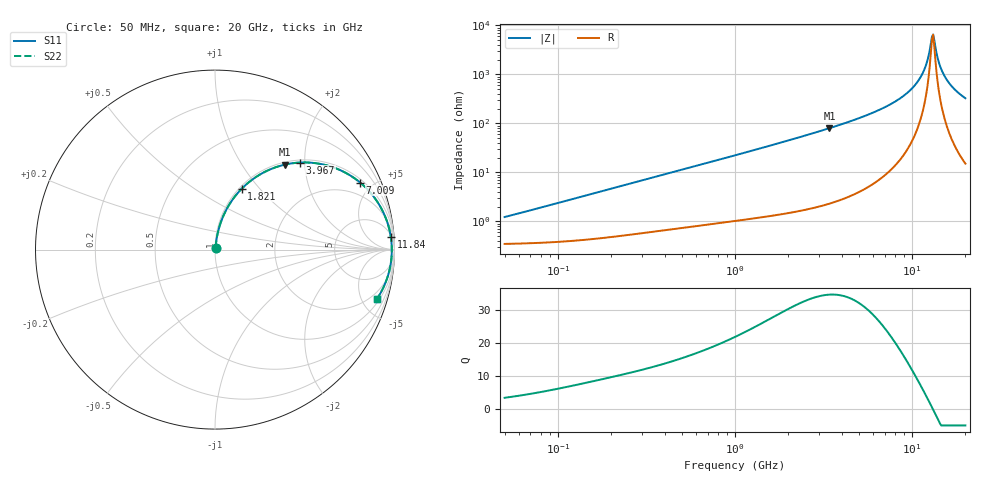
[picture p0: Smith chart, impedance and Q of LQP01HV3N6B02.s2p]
!Murata Part Number: LQP01HV3N6B02
!These Parameters are Measured in Series Mode Connection
!  o--[Z]--o
!Port1  Port2
!  o-------o
!Freq. Start=50[MHz] Stop=20[GHz], 401[Steps]
# Hz S RI R 50
!Freq.(Hz) S11(Real) S11(Imag) S21(Real) S21(Imag) S12(Real) S12(Imag) S22(Real) S22(Imag)
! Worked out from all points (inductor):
!   401 points, 50 MHz to 20 GHz, reference 50 ohm
!   read as one part in series: L = 3.72 nH near 51.52 MHz
!   highest Q = 34.7 at 3.415 GHz (marker M1), where L = 3.7 nH
!   self-resonance near 12.95 GHz
!   S11 on the Smith chart (normalised r, x): 50 MHz: 1.01, +0.02; 1.821 GHz: 1.03, +0.81; 3.967 GHz: 1.05, +1.89; 7.009 GHz: 1.17, +4.24; 11.84 GHz: 7, +27; 20 GHz: 1.30, -6.48
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5e7  0.00357 0.0116  0.9964 -0.0116  0.9964 -0.0116  0.00357 0.0116
1.364002e8  0.0051 0.0313  0.9949 -0.0313  0.9949 -0.0313  0.0051 0.0313
3.721004e8  0.0132 0.0824  0.9868 -0.0824  0.9868 -0.0824  0.0132 0.0824
1e9  0.0554 0.207  0.9446 -0.207  0.9446 -0.207  0.0554 0.207
1.820564e9  0.1492 0.3395  0.8508 -0.3395  0.8508 -0.3395  0.1492 0.3395
2.728004e9  0.283 0.4358  0.717 -0.4358  0.717 -0.4358  0.283 0.4358
3.415248e9  0.3901 0.4736  0.6099 -0.4736  0.6099 -0.4736  0.3901 0.4736
3.967106e9  0.4732 0.485  0.5268 -0.485  0.5268 -0.485  0.4732 0.485
5.273168e9  0.6453 0.4627  0.3547 -0.4627  0.3547 -0.4627  0.6453 0.4627
7.009217e9  0.8088 0.3734  0.1912 -0.3734  0.1912 -0.3734  0.8088 0.3734
7.442007e9  0.8387 0.3464  0.1613 -0.3464  0.1613 -0.3464  0.8387 0.3464
1.004137e10  0.9507 0.1776  0.0493 -0.1776  0.0493 -0.1776  0.9507 0.1776
1.098561e10  0.9697 0.1192  0.0303 -0.1192  0.0303 -0.1192  0.9697 0.1192
1.183995e10  0.9798 0.069  0.0202 -0.069  0.0202 -0.069  0.9798 0.069
1.220001e10  0.9824 0.0486  0.0176 -0.0486  0.0176 -0.0486  0.9824 0.0486
1.276073e10  0.9846 0.0179  0.0154 -0.0179  0.0154 -0.0179  0.9846 0.0179
1.314879e10  0.9851 -0.00257  0.0149 0.00257  0.0149 0.00257  0.9851 -0.00257
1.334722e10  0.9849 -0.0128  0.0151 0.0128  0.0151 0.0128  0.9849 -0.0128
1.438523e10  0.9811 -0.064  0.0189 0.064  0.0189 0.064  0.9811 -0.064
1.527346e10  0.9743 -0.1045  0.0257 0.1045  0.0257 0.1045  0.9743 -0.1045
1.721783e10  0.9504 -0.1831  0.0496 0.1831  0.0496 0.1831  0.9504 -0.1831
2e10  0.9028 -0.274  0.0972 0.274  0.0972 0.274  0.9028 -0.274
